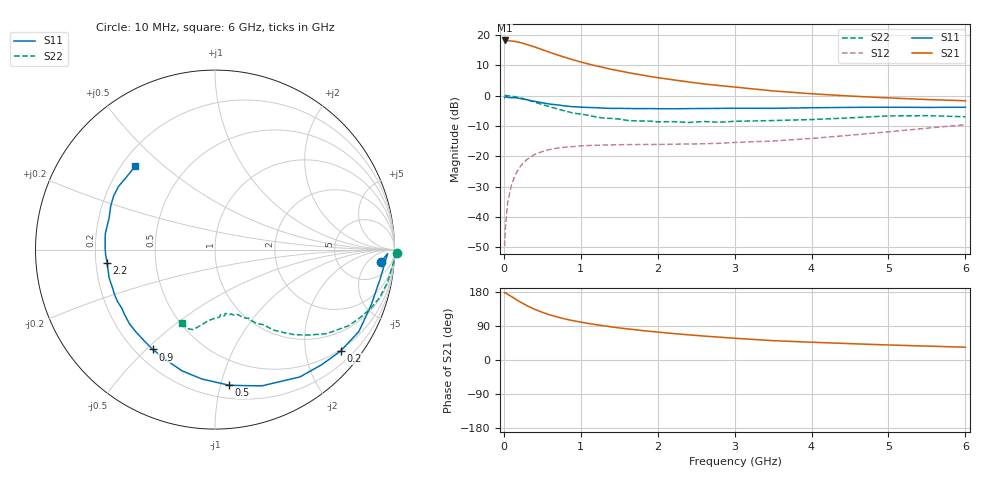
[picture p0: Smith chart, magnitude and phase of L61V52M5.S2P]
!  INFINEON TECHNOLOGIES Small Signal Semiconductors
! BFR380L3 , Si-NPN RF-Transistor in TSLP-3-1
!  Vce=1.5 V,  Ic=2.5 mA
! Common Emitter S-Parameters:  07. March 2005
#  GHz  S  MA  R  50
! f  S11  S21  S12  S22
! GHz  Mag  Ang  Mag  Ang  Mag  Ang  Mag  Ang
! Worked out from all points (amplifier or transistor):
!   36 points, 10 MHz to 6 GHz, reference 50 ohm
!   highest |S21| = 18.2 dB at 10 MHz (marker M1)
!   |S21| within 3 dB of that: start of sweep to 496.5 MHz
!   unconditionally stable (mu >= 1): 2.696 GHz to 4.732 GHz
!   at 250 MHz: K = 0.11, MSG = 19.8 dB, |S12| = -22.3 dB
!   at 1.4 GHz: K = 0.60, MSG = 12.4 dB, |S12| = -16.3 dB
!   at 6 GHz: K = 0.92, MSG = 3.9 dB, |S12| = -9.6 dB
!   S11 on the Smith chart (normalised r, x): 10 MHz: 13, -13; 200 MHz: 0.47, -2.76; 500 MHz: 0.30, -1.07; 900 MHz: 0.27, -0.52; 2.2 GHz: 0.25, -0.06; 6 GHz: 0.25, +0.40
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0.01  0.9251 -4.4  8.089 177.1  0.0033 89.0  1.015 -1.1
0.02  0.9622 -1.3  8.071 177.8  0.0065 87.1  1.004 -2.4
0.05  0.9347 -10.0  8.058 173.5  0.0174 86.1  0.992 -5.5
0.1  0.9232 -19.6  7.909 167.2  0.0339 79.7  0.9776 -10.9
0.15  0.9223 -29.7  7.787 160.7  0.0498 74.2  0.9555 -16.3
0.2  0.8996 -38.9  7.536 154.5  0.064 69.4  0.9265 -20.8
0.3  0.8527 -56.3  6.937 143.4  0.0882 60.5  0.8566 -29.7
0.4  0.8027 -71.1  6.324 133.8  0.1069 53.1  0.7794 -36.9
0.5  0.7602 -84.0  5.706 125.9  0.1194 47.7  0.7109 -42.0
0.6  0.7246 -95.8  5.138 118.8  0.1296 42.9  0.6523 -46.7
0.7  0.7001 -105.2  4.654 113.3  0.1367 39.7  0.6013 -50.3
0.8  0.673 -113.7  4.246 108.1  0.1412 37.3  0.5557 -53.9
0.9  0.6554 -121.9  3.878 103.7  0.1446 34.9  0.5156 -56.1
1.1  0.6362 -133.6  3.314 96.3  0.1505 32.6  0.4721 -60.6
1.5  0.6153 -152.2  2.553 84.6  0.1549 30.6  0.4094 -67.6
1.9  0.6107 -165.1  2.063 75.6  0.1561 31.6  0.3794 -74.3
2.2  0.6058 -172.8  1.817 69.9  0.1582 33.6  0.372 -76.8
2.6  0.6123 179.0  1.556 63.2  0.1606 37.5  0.3735 -82.0
3.5  0.6162 163.0  1.193 51.0  0.1785 47.0  0.3877 -92.3
4.5  0.6384 152.4  0.982 43.2  0.2219 57.3  0.4289 -100.6
5.5  0.6377 140.7  0.86 36.7  0.29 61.4  0.4662 -109.1
6  0.6427 133.9  0.821 33.8  0.3315 61.1  0.4473 -113.9
